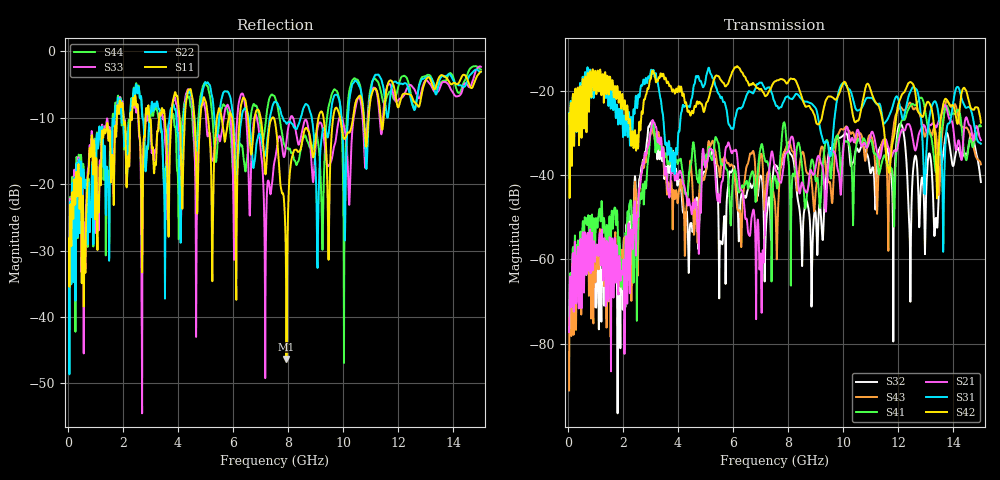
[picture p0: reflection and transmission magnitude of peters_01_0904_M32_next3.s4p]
# MHZ S RI R 50.00
! FREQ  S11  S12  S13  S14
!  S21  S22  S23  S24
!  S31  S32  S33  S34
!  S41  S42  S43  S44
!  REAL  IMAG  REAL  IMAG  REAL  IMAG  REAL  IMAG
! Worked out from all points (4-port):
!   1496 points, 50 MHz to 15 GHz, reference 50 ohm
!   strongest paths, dB at 50 MHz, 3.79 GHz, 7.53 GHz, 11.27 GHz, 15 GHz:
!     S42: -25.4, -20.0, -17.7, -23.3, -27.5
!     S31: -25.2, -38.7, -22.9, -23.0, -32.5
!     S21: -77.3, -38.6, -38.2, -35.2, -31.6
!     S41: -76.8, -34.2, -40.3, -38.4, -28.4
!     S43: -91.1, -45.1, -46.9, -41.3, -37.4
!     S32: -75.2, -35.1, -37.6, -34.9, -41.6
!   lowest |S11| = -46.3 dB at 7.94 GHz (marker M1), VSWR 1.01, Z = 50.4 - j0.317 ohm
!   |S11| at or under -10 dB: start of sweep to 1.783 GHz; 7.472 GHz to 9.106 GHz (1.634 GHz wide, 19.7 % of centre); 9.887 GHz to 10.36 GHz (471.9 MHz wide, 4.66 % of centre)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
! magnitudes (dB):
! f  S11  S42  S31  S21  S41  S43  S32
! 50 MHz  -28.2  -25.4  -25.2  -77.3  -76.8  -91.1  -75.2
! 1.86 GHz  -9.0  -22.5  -24.8  -60.3  -56.0  -65.3  -60.3
! 3.03 GHz  -11.6  -16.6  -14.9  -28.9  -28.9  -29.7  -27.4
! 7.02 GHz  -10.4  -19.5  -17.9  -61.9  -33.0  -34.9  -40.2
! 7.94 GHz  -46.3  -18.1  -21.4  -34.6  -31.7  -33.1  -33.6
! 8.86 GHz  -14.8  -24.4  -23.0  -39.3  -36.3  -41.8  -68.0
! 15 GHz  -3.1  -27.5  -32.5  -31.6  -28.4  -37.4  -41.6
